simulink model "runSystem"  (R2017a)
settings: Solver=VariableStepAuto  StartTime=0.0  StopTime=2  RelTol=1e-3
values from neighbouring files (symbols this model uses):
  baud = 250000    [MISOcontrol.m]    (also in MISO_demo.m; runSteptest.m; SISOcontrol.m; init.m)
  com = 'COM4'    [MISOcontrol.m]    (also in MISO_demo.m; runSteptest.m; SISOcontrol.m; init.m)
  fTf = 0.1    [MISOcontrol.m]    (also in MISO_demo.m; runSteptest.m; SISOcontrol.m; init.m)
  fTl = 0.05    [MISOcontrol.m]    (also in MISO_demo.m; runSteptest.m; SISOcontrol.m; init.m)
  fTt = 0.05    [MISOcontrol.m]    (also in MISO_demo.m; runSteptest.m; SISOcontrol.m; init.m)
  stepBulb = 0    [MISOcontrol.m]    (also in MISO_demo.m; runSteptest.m; SISOcontrol.m; steadyState.m = 0.5)
  stepFan = 0    [MISOcontrol.m]    (also in MISO_demo.m; runSteptest.m; SISOcontrol.m; steadyState.m = 0.2)
  stepLed = 0    [MISOcontrol.m]    (also in MISO_demo.m; runSteptest.m = 1; SISOcontrol.m; steadyState.m = 0.5)
  t_step = 0    [MISOcontrol.m]    (also in MISO_demo.m = 20; runSteptest.m = 10; SISOcontrol.m = 10; steadyState.m)
  Ts = 0.1    [identification.m]    (also in MISOcontrol.m; MISO_demo.m; runSteptest.m; SISOcontrol.m)
libraries: tom_lib x1

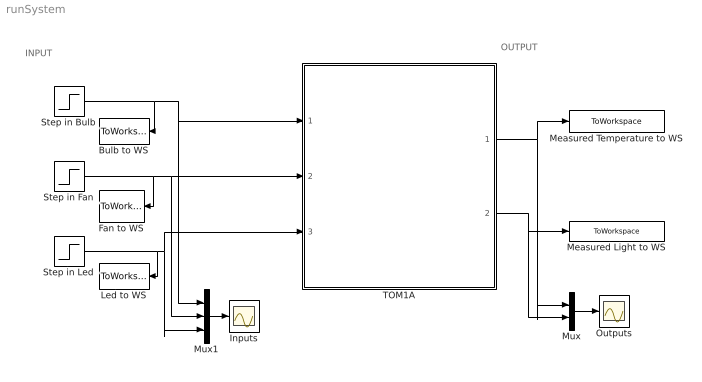
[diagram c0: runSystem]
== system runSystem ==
  note: INPUT
  note: OUTPUT
  Bulb to WS : ToWorkspace  VariableName=bulbInput  SampleTime=-1
  Fan to WS : ToWorkspace  VariableName=fanInput  SampleTime=-1
  Inputs : Scope
  Led to WS : ToWorkspace  VariableName=ledInput  SampleTime=-1
  Measured Light to WS : ToWorkspace  VariableName=LightIntensity  SampleTime=-1
  Measured Temperature to WS : ToWorkspace  VariableName=Temperature  SampleTime=-1
  Mux : Mux  Inputs=2
  Mux1 : Mux  Inputs=3
  Outputs : Scope
  Step in Bulb : Step  Time=t_step  After=stepBulb  SampleTime=Ts
  Step in Fan : Step  Time=t_step  After=stepFan  SampleTime=Ts
  Step in Led : Step  Time=t_step  After=stepLed  SampleTime=Ts
  TOM1A : Subsystem
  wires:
  Mux1/1 -> Inputs/1
  Mux/1 -> Outputs/1
  TOM1A/2(Light Intensity) -> Mux/2, Measured Light to WS/1
  TOM1A/1(Temperature) -> Mux/1, Measured Temperature to WS/1
  Step in Bulb/1 -> Bulb to WS/1, Mux1/1, TOM1A/1(Bulb)
  Step in Fan/1 -> Fan to WS/1, Mux1/2, TOM1A/2(Fan)
  Step in Led/1 -> Led to WS/1, Mux1/3, TOM1A/3(LED)

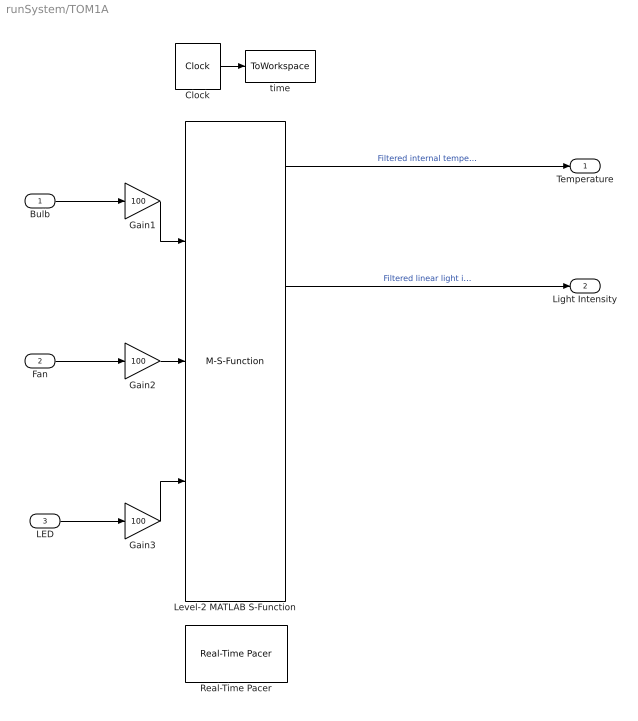
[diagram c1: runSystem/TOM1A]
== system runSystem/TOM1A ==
  Bulb : Inport
  Fan : Inport  Port=2
  LED : Inport  Port=3
  Clock : Clock
  Gain1 : Gain  Gain=100
  Gain2 : Gain  Gain=100
  Gain3 : Gain  Gain=100
  Level-2 MATLAB S-Function : M-S-Function  FunctionName=tom1ar8  Parameters=Ts,com,baud,fTt,fTl,fTf
  Real-Time Pacer : tom_lib/Real-Time Pacer  simTimePerRealTime=1
  time : ToWorkspace  VariableName=time  SampleTime=-1
  Temperature : Outport
  Light Intensity : Outport  Port=2
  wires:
  LED/1 -> Gain3/1
  Fan/1 -> Gain2/1
  Bulb/1 -> Gain1/1
  Level-2 MATLAB S-Function/8 -> ?  "Filtered logaritmic light intensity"
  Level-2 MATLAB S-Function/12 -> ?  "Fan current"
  Level-2 MATLAB S-Function/6 -> Light Intensity/1  "Filtered linear light intensity"
  Level-2 MATLAB S-Function/10 -> ?  "Bulb current"
  Level-2 MATLAB S-Function/4 -> ?  "Filtered external temperature"
  Level-2 MATLAB S-Function/14 -> ?  "Fan filtered  rpm"
  Level-2 MATLAB S-Function/9 -> ?  "Derivate of logaritmic light intensity"
  Level-2 MATLAB S-Function/2 -> Temperature/1  "Filtered internal temperature"
  Gain3/1 -> Level-2 MATLAB S-Function/3
  Level-2 MATLAB S-Function/5 -> ?  "Derivate of external temperature"
  Level-2 MATLAB S-Function/15 -> ?  "Derivate of fan rpm"
  Level-2 MATLAB S-Function/1 -> ?  "Board temperature"
  Clock/1 -> time/1
  Level-2 MATLAB S-Function/3 -> ?  "Derivative of internal temperature"
  Gain1/1 -> Level-2 MATLAB S-Function/1
  Level-2 MATLAB S-Function/16 -> ?  "Count of fan rpm"
  Level-2 MATLAB S-Function/11 -> ?  "Bulb voltage"
  Level-2 MATLAB S-Function/7 -> ?  "Derivate of linear light intensity"
  Gain2/1 -> Level-2 MATLAB S-Function/2
  Level-2 MATLAB S-Function/13 -> ?  "Fan voltage"
